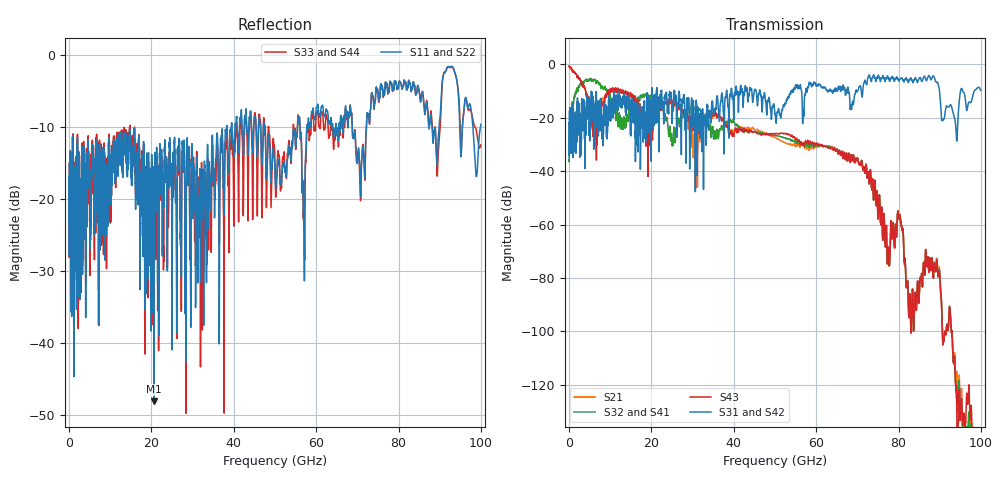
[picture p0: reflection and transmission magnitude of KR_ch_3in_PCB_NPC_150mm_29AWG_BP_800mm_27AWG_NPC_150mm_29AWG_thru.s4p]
# GHz S RI R 45
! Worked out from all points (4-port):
!   4000 points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, 25 MHz to 100 GHz, reference 45 ohm
!   strongest paths, dB at 25 MHz, 25.02 GHz, 50.02 GHz, 75.03 GHz, 100 GHz:
!     S31: -22.2, -20.9, -18.6, -4.1, -9.7
!     S42: -22.2, -20.8, -18.7, -4.1, -9.8
!     S43: -0.7, -13.5, -26.0, -57.1, -137.5
!     S32: -35.9, -29.9, -26.6, -57.2, -145.1
!     S41: -35.9, -29.8, -26.6, -57.2, -145.1
!     S21: -0.7, -13.6, -27.4, -57.2, -155.3
!   lowest |S11| = -48.1 dB at 20.65 GHz (marker M1), VSWR 1.01, Z = 45.2 + j0.299 ohm
!   |S11| at or under -10 dB: start of sweep to 38.28 GHz; 47.38 GHz to 55.47 GHz (8.097 GHz wide, 15.7 % of centre); 68.76 GHz to 72.21 GHz (3.448 GHz wide, 4.89 % of centre)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
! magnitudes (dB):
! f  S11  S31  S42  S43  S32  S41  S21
! 25 MHz  -17.4  -22.2  -22.2  -0.7  -35.9  -35.9  -0.7
! 3.8 GHz  -19.7  -23.4  -23.4  -8.6  -6.1  -6.1  -8.6
! 20.65 GHz  -48.1  -15.5  -15.5  -22.4  -13.3  -13.3  -20.5
! 64.12 GHz  -10.7  -10.1  -10.2  -32.2  -31.8  -31.8  -31.4
! 80.22 GHz  -3.7  -5.8  -5.9  -57.4  -57.5  -57.5  -57.5
! 82.25 GHz  -4.6  -5.9  -5.9  -81.1  -81.1  -81.1  -81.1
! 100 GHz  -9.7  -9.7  -9.8  -137.5  -145.1  -145.1  -155.3
